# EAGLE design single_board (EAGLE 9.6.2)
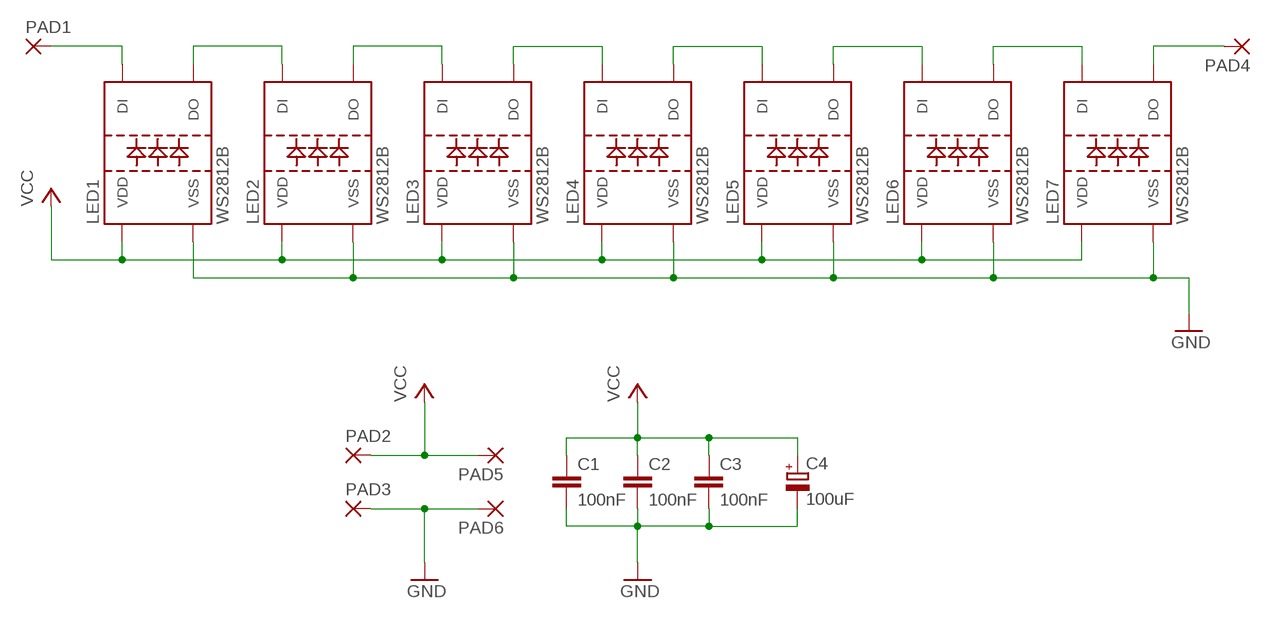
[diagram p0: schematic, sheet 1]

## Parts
C1  100nF  C-EUC0805  [C0805]
C2  100nF  C-EUC0805  [C0805]
C3  100nF  C-EUC0805  [C0805]
C4  100uF  CPOL-EUUD-6,3X7,7  [UD-6,3X7,7_NICHICON]
LED1  WS2812B  [WS2812B]
LED2  WS2812B  [WS2812B]
LED3  WS2812B  [WS2812B]
LED4  WS2812B  [WS2812B]
LED5  WS2812B  [WS2812B]
LED6  WS2812B  [WS2812B]
LED7  WS2812B  [WS2812B]
PAD1  SMD5  [SMD2,54-5,08]
PAD2  SMD5  [SMD2,54-5,08]
PAD3  SMD5  [SMD2,54-5,08]
PAD4  SMD5  [SMD2,54-5,08]
PAD5  SMD5  [SMD2,54-5,08]
PAD6  SMD5  [SMD2,54-5,08]

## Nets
GND: C1.2 C2.2 C3.2 C4.- LED1.3(VSS) LED2.3(VSS) LED3.3(VSS) LED4.3(VSS) LED5.3(VSS) LED6.3(VSS) LED7.3(VSS) PAD3.1(P) PAD6.1(P)
N$1: LED2.2(DO) LED3.4(DI)
N$2: LED1.2(DO) LED2.4(DI)
N$3: LED3.2(DO) LED4.4(DI)
N$4: LED4.2(DO) LED5.4(DI)
N$5: LED5.2(DO) LED6.4(DI)
N$6: LED6.2(DO) LED7.4(DI)
N$7: LED1.4(DI) PAD1.1(P)
N$10: LED7.2(DO) PAD4.1(P)
VCC: C1.1 C2.1 C3.1 C4.+ LED1.1(VDD) LED2.1(VDD) LED3.1(VDD) LED4.1(VDD) LED5.1(VDD) LED6.1(VDD) LED7.1(VDD) PAD2.1(P) PAD5.1(P)

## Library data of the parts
C1-C3 = rcl:C-EU: CAPACITOR, European symbol; SPICEPREFIX: C
C4 = rcl:CPOL-EU: POLARIZED CAPACITOR, European symbol; SPICEPREFIX: C
LED1-LED7 = WS2812:WS2812B
PAD1-PAD6 = wirepad:SMD5: SMD PAD

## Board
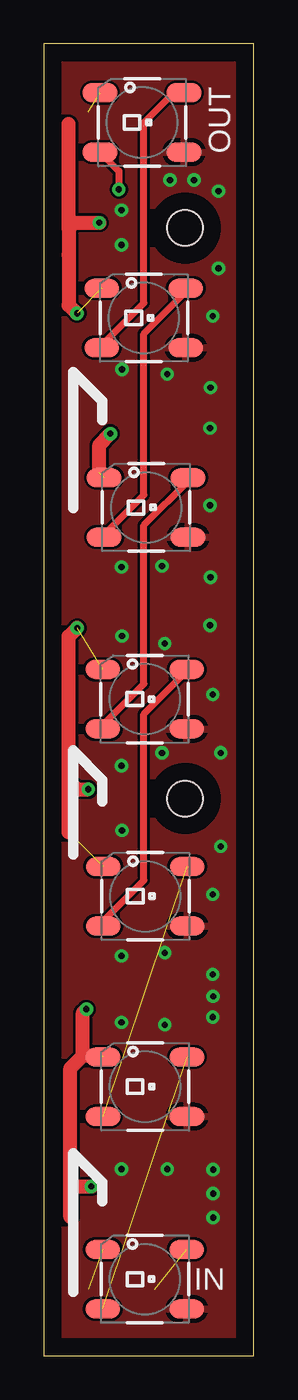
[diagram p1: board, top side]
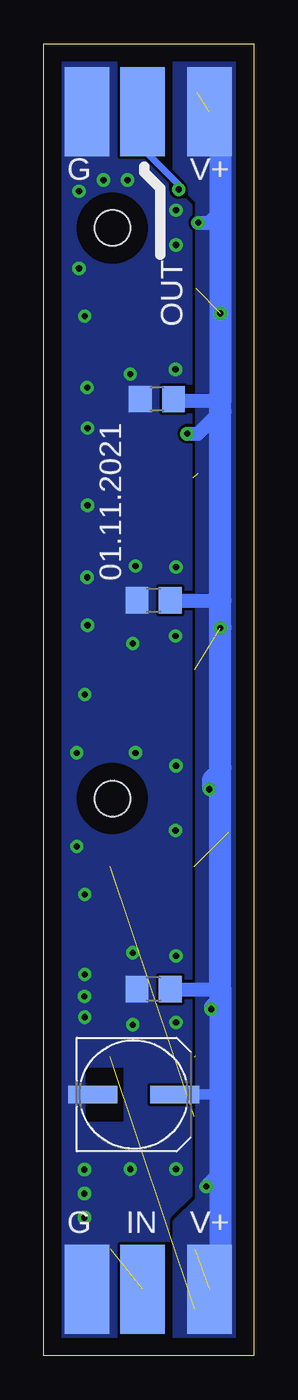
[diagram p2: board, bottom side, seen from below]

Size 12 x 75 mm. Coordinates in mm from the lower left corner, seen from the top.
Outline: 0,0 12,0 12,75 0,75 0,0
Copper layers (1*16): Top 0.035mm / dielectric 1.5mm / Bottom 0.035mm
Design rules "default *": minimum track width 6mil, minimum drill 0.35mm, track to track 6mil, track to pad 6mil, pad to pad 6mil, via to via 6mil, smd to smd 6mil, copper to edge 40mil, drill to drill 6mil, minimum pad ring 10mil, minimum via ring 8mil, stop-mask expansion 4mil, vias tented up to drill 16mil, thermal gap 10mil
Holes 2.03 mm at 8.08,64.47 8.08,31.85
bRestrict: area 7.5,13.4 to 9.6,16.5

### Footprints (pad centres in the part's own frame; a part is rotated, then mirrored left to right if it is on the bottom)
C0805 = smd 1.3 x 1.5: 1 -0.95,0; 2 0.95,0
UD-6,3X7,7_NICHICON = smd 2.8 x 1: + 2.35,0; - -2.35,0
WS2812B = smd 2 x 1.1: 1 -2.4,1.7; 2 -2.4,-1.7; 3 2.4,-1.7; 4 2.4,1.7
SMD2,54-5,08 = smd 2.54 x 5.08: 1 0,0

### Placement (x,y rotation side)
C1  5.71,20.95 180 bottom
C2  5.71,43.18 180 bottom
C3  5.53,54.69 180 bottom
C4  6.86,14.94 0 bottom
LED1  5.78,4.38 0 top
LED2  5.79,15.38 0 top
LED3  5.8,26.27 0 top
LED4  5.77,37.54 0 top
LED5  5.85,48.49 0 top
LED6  5.71,59.33 0 top
LED7  5.62,70.5 0 top
PAD1  6.35,3.81 0 bottom
PAD2  2.54,3.81 0 bottom
PAD3  9.53,3.81 0 bottom
PAD4  6.35,71.12 0 bottom
PAD5  2.54,71.12 0 bottom
PAD6  9.53,71.12 180 bottom

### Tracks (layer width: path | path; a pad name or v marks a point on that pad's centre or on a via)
GND  (via drill 0.35)
  other vias: 9.68,10.64 9.65,21.79 10.11,34.47 9.53,44.5 9.53,55.35 8.59,67.21 4.45,33.73 4.45,10.67 4.45,19.05 4.45,22.86 4.45,45.09 4.45,63.5 9.68,7.9 9.68,9.27 9.98,66.57 9.68,20.55 9.65,59.44 9.5,48.62 9.65,37.8 9.65,26.37 7.06,10.67 9.65,19.35 10.11,29.11 9.5,41.76 9.5,53.04 7.21,67.21 4.47,56.39 4.47,41.15 4.47,30.02 4.45,65.48 9.98,62.15 6.76,34.47 6.91,40.72 6.91,23.04 6.76,45.14 7.06,56.11 6.91,18.92
  pour Bottom (rank 4, no thermals): -0.64,76.2 13.34,76.2 13.34,-3.17 -3.17,-3.17 -3.17,74.93 -1.91,76.2
  pour Top: -1.27,76.2 12.7,76.2 13.34,75.56 13.34,-3.81 -2.54,-3.81 -2.54,74.93
N$1  (1 unrouted)
N$2  (1 unrouted)
N$3
  Top 0.406: LED3.2 3.4,24.87 5.71,27.18 5.71,36.68 8.17,39.13 LED4.4
N$4
  Top 0.406: LED4.2 3.37,36.06 5.71,38.41 5.71,47.47 8.25,50.01 LED5.4
N$5
  Top 0.406: LED5.2 3.45,46.94 5.71,49.21 5.71,58.42 8.12,60.82 LED6.4
N$6
  Top 0.406: LED6.2 3.31,57.78 5.71,60.18 5.71,70.48 7.43,72.2 LED7.4
N$7  (1 unrouted)
N$10  (via drill 0.35)
  Top 0.406: LED7.2 4.29,67.73 v4.29,66.67
  Bottom 0.406: v4.29,66.67 4.29,66.95 6.35,69.01 PAD4.1
VCC  (via drill 0.35)  (7 unrouted)
  Top 0.813: 1.53,7.92 1.53,9.5 | 1.53,9.5 1.53,16.44 2.23,17.14 | 3.33,17.14 2.23,17.14 | 1.53,9.5 1.7,9.68 v2.72,9.68 | 1.42,29.94 1.42,32.87 | 1.42,32.87 1.42,37.29 1.42,41.12 v1.91,41.6 | 1.42,32.87 1.91,32.38 v2.54,32.38 | 3.17,50.47 3.17,52.07 v3.81,52.7 | 1.42,64.44 1.42,62.92 1.42,60.05 1.88,59.59 v1.91,59.59 | 1.42,64.44 1.42,70.4 | 1.42,64.44 1.75,64.77 v3.17,64.77 | 2.23,17.14 2.23,19.61 v2.44,19.81
  Bottom 0.61: C4.+ 1.91,14.94
  Bottom 0.813: C3.1 4.5,54.61 1.91,54.61 | C2.1 1.91,43.18 | C1.1 1.91,20.95 | v2.72,9.68 2.23,10.16 1.91,10.16 | v2.54,32.38 2.54,33.02 1.91,33.66 | v3.81,52.7 3.17,52.7 1.91,53.98 | v3.17,64.77 2.54,64.77 1.91,65.41 | v2.44,19.81 2.44,19.96 2.29,20.12 1.91,20.12
  Bottom 1.27: PAD2.1 1.91,4.45 1.91,10.16 1.91,14.94 1.91,20.12 1.91,20.95 1.91,33.66 v1.91,41.6 1.91,43.18 1.91,53.98 1.91,54.61 v1.91,59.59 1.91,65.41 1.91,70.48 PAD5.1
  pour Bottom (rank 3, no thermals): -1.27,76.2 4.45,76.2 4.45,67.31 3.17,66.04 3.17,8.89 4.45,7.62 4.45,-1.27 -1.27,-1.27

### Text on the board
tNames: OUT | IN
bNames: V+ | G | OUT | 01.11.2021 | V+ | IN | G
